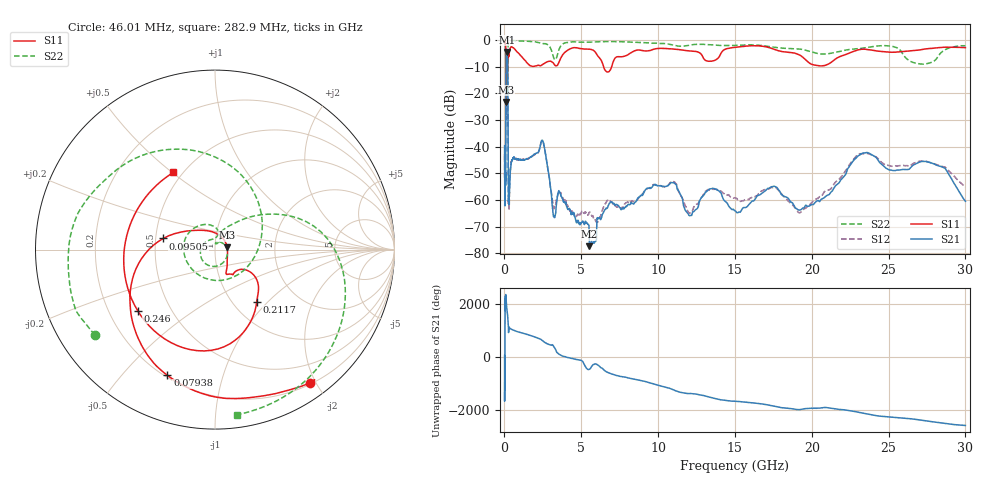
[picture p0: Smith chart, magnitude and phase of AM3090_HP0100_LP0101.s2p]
! Date/Time: Thu, Feb 28, 2019 1:57 PM
! Network Analyzer: Agilent Technologies E8364B Rev: A.07.50.67
! Sweep from 0.010 to 30.000 GHz, 1601 Points, Sweep Type: LOG
! Power Supply: 5.023 V, 0.002 A
# Hz S DB R 50
!freq MagS11 AngS11 MagS21 AngS21 MagS12 AngS12 MagS22 AngS22
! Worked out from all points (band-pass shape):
!   1601 points, 10 MHz to 30 GHz, reference 50 ohm
!   highest |S21| = -4.47 dB at 146.9 MHz (marker M1); lowest = -77.4 dB at 5.528 GHz (marker M2)
!   |S21| within 3 dB of the highest: 105.3 MHz to 201.8 MHz (96.5 MHz wide, 62.8 % of centre)
!   lowest |S11| = -23.2 dB at 103.5 MHz (marker M3), VSWR 1.15, Z = 57.3 + j1.41 ohm
!   |S11| at or under -10 dB: 94.64 MHz to 203.1 MHz (108.5 MHz wide, 72.9 % of centre); 6.455 GHz to 6.978 GHz (523.7 MHz wide, 7.8 % of centre)
!   |S22| runs from -29.8 to -0.2 dB; largest |S21 - S12| = 0.016
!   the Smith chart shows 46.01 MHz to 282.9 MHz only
!   S11 on the Smith chart (normalised r, x): 46.01 MHz: 0.21, -1.91; 79.38 MHz: 0.21, -0.67; 95.05 MHz: 0.55, +0.07; 211.7 MHz: 1.28, -0.86; 246 MHz: 0.32, -0.31; 282.9 MHz: 0.45, +0.50
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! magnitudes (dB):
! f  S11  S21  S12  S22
! 10 MHz  -0.3  -39.6  -44.9  -0.6
! 38.04 MHz  -0.5  -60.7  -58.4  -1.4
! 46.01 MHz  -0.8  -51.6  -53.6  -1.7
! 79.38 MHz  -2.5  -48.9  -47.0  -4.9
! 95.05 MHz  -10.6  -16.1  -16.0  -15.3
! 103.5 MHz  -23.2  -8.2  -8.2  -15.2
! 144.7 MHz  -16.0  -4.5  -4.4  -24.2
! 146.9 MHz  -15.9  -4.5  -4.4  -23.6
! 211.7 MHz  -8.6  -10.7  -10.7  -13.1
! 246 MHz  -5.2  -53.2  -54.9  -1.5
! 282.9 MHz  -6.2  -61.8  -60.1  -0.6
! 550.5 MHz  -2.9  -44.3  -44.2  -0.2
! 2.084 GHz  -9.7  -42.4  -42.7  -0.7
! 2.507 GHz  -9.1  -38.0  -38.1  -1.3
! 3.204 GHz  -8.8  -66.0  -62.3  -6.7
! 3.613 GHz  -7.4  -57.3  -57.4  -2.7
! 5.528 GHz  -3.4  -77.4  -64.7  -0.8
! 7.926 GHz  -5.8  -62.3  -61.0  -0.7
! 10.76 GHz  -3.3  -54.0  -53.8  -1.6
! 19.41 GHz  -6.4  -63.1  -63.9  -3.6
! 23.48 GHz  -3.5  -42.3  -42.5  -2.9
! 30 GHz  -2.9  -60.5  -55.2  -2.1
